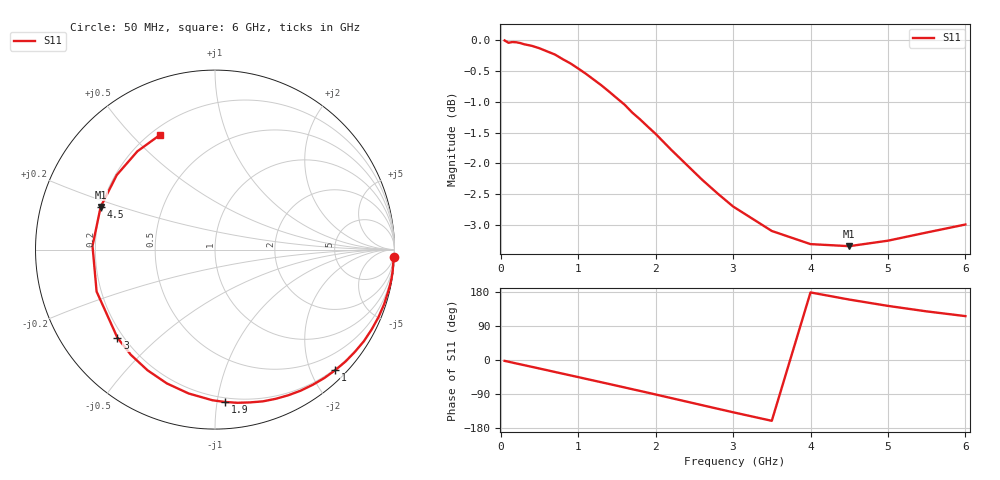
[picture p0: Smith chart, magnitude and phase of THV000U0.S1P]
! SIEMENS Discrete & RF Semiconductors
! BAS70
! Si Schottky Diode in SOT23
! VR = 0 V
! S-Parameters:  February  1997
# GHz  S  MA  R  50
!  f  S11
! GHz  MAG  ANG
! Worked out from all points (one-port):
!   34 points, 50 MHz to 6 GHz, reference 50 ohm
!   lowest |S11| = -3.3 dB at 4.5 GHz (marker M1), VSWR 5.25, Z = 9.82 + j8.7 ohm
!   |S11| at or under -10 dB: nowhere
!   S11 on the Smith chart (normalised r, x): 50 MHz: 0, -50; 1 GHz: 0.18, -2.40; 1.9 GHz: 0.17, -1.05; 3 GHz: 0.18, -0.37; 4.5 GHz: 0.20, +0.17; 6 GHz: 0.24, +0.60
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0.05  1 -2.3
0.25  0.9952 -11.3
0.4  0.99 -18.0
0.5  0.9855 -22.5
0.6  0.9797 -27.0
0.7  0.974 -31.6
0.8  0.9656 -36.1
0.9  0.9579 -40.6
1  0.9488 -45.1
1.1  0.9395 -49.7
1.3  0.9194 -58.8
1.4  0.9085 -63.3
1.5  0.8974 -67.9
1.6  0.8865 -72.5
1.8  0.8625 -81.7
1.9  0.8507 -86.3
2  0.8394 -91.0
2.2  0.8149 -100.4
2.4  0.7923 -109.8
2.6  0.7704 -119.2
2.8  0.7507 -128.6
3  0.7327 -137.9
3.5  0.6998 -160.5
4  0.6828 178.3
4.5  0.6802 159.5
5  0.6872 142.8
5.5  0.6978 128.3
6  0.7083 115.8
